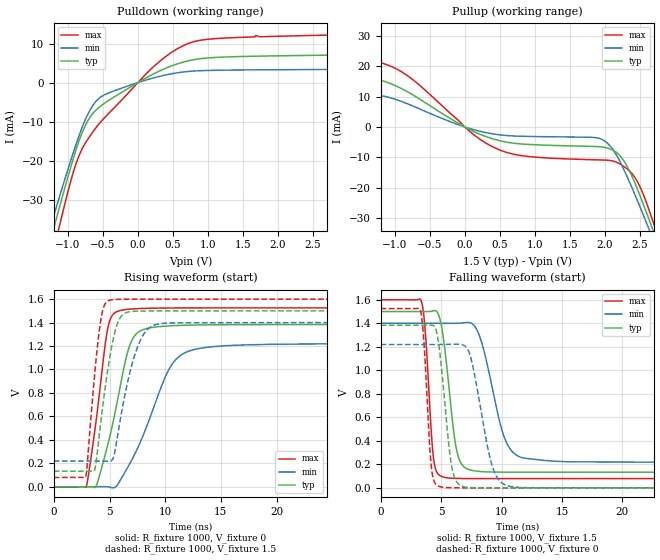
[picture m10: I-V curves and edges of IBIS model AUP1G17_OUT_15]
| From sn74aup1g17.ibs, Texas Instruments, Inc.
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[Model]   AUP1G17_OUT_15
Model_type  Output
Vref =   0
Rref =   1E6
Cref =   30p
Vmeas =   0.75
| variable   typ   min   max
C_comp   2.88pF   2.08pF   4.08pF
| C_pullup   3.12pF   2.08pF   4.08pF
| C_pulldown   2.65pF   2.24pF   3.14pF
[Temperature Range]   40   100   -40
| Ambient temperature   25   85   -40
[Voltage range]   1.5   1.4   1.6
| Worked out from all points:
|   slope of the pulldown table from 0 to 0.225 V, typ, clamps not added: 101 ohm
|   slope of the pullup table from 0 to 0.225 V, typ, clamps not added: 90.4 ohm
|   rising waveform, R_fixture 1000, V_fixture 0: 20-80 % time 1.89ns typ, 3.12ns min, 1.2ns max; typ from 0 V to 1.38 V
|   falling waveform, R_fixture 1000, V_fixture 1.5: 20-80 % time 888ps typ, 1.59ns min, 538ps max; typ from 1.5 V to 0.133 V
|   rising waveform, R_fixture 1000, V_fixture 1.5: 20-80 % time 1.22ns typ, 1.65ns min, 879ps max; typ from 0.133 V to 1.5 V
|   falling waveform, R_fixture 1000, V_fixture 0: 20-80 % time 801ps typ, 1.33ns min, 499ps max; typ from 1.38 V to 0 V
[Pulldown]
| AUP1G17_OUT_15
|   Voltage   I(typ)   I(min)   I(max)
-3.6V     -206.1mA   -188.4mA   -227.8mA
-1.265V   -41.59mA   -37.94mA   -47.65mA
-1.21V    -37.9mA    -34.62mA   -43.48mA
-1.11V    -31.29mA   -28.67mA   -36mA
-945mV    -20.84mA   -19.21mA   -24.37mA
-855mV    -15.7mA    -14.39mA   -19.43mA
-720mV    -9.972mA   -8.297mA   -14.65mA
-570mV    -6.595mA   -4.269mA   -10.91mA
260mV     2.544mA    1.373mA    4.642mA
810mV     5.906mA    2.979mA    10.53mA
1.685V    6.762mA    3.268mA    12.01mA
7.2V      7.827mA    3.609mA    13.77mA
[Pullup]
| AUP1G17_OUT_15
|   Voltage   I(typ)   I(min)   I(max)
-3.6V     29.66mA    17.95mA    40.7mA
-2.925V   22.54mA    13.64mA    31.9mA
-2.13V    15.77mA    9.503mA    23.16mA
-1.025V   13.91mA    9.322mA    19.64mA
130mV     -1.525mA   -910.1uA   -2.565mA
590mV     -4.979mA   -2.819mA   -8.32mA
1.925V    -6.506mA   -3.765mA   -10.85mA
2.175V    -8.513mA   -9.57mA    -11.67mA
2.395V    -16.55mA   -20.31mA   -15.49mA
2.615V    -29.32mA   -32.63mA   -26.15mA
2.72V     -35.89mA   -38.74mA   -33.2mA
7.2V      -352.6mA   -330.3mA   -379.5mA
[Ramp]
| AUP1G17_OUT_15
| variable   typ   min   max
dV/dt_r   0.83/1.91E-09   0.74/3.15E-09   0.92/1.20E-09
dV/dt_f   0.83/8.95E-10   0.71/1.60E-09   0.92/5.43E-10
R_load = 1000
[Rising Waveform]
| AUP1G17_OUT_15
R_fixture =   1000
C_fixture =   0
L_fixture =   0
V_fixture =   0
V_fixture_min = 0
V_fixture_max = 0
|   Time   V(typ)   V(min)   V(max)
0s        16.57nV    92.2nV     986.7pV
2.925ns   299.7uV    -18.59uV   4.96mV
3.795ns   5.632mV    236.3uV    562.4mV
4.78ns    335.2mV    269.9uV    1.318V
5.655ns   706.7mV    9.617mV    1.493V
6.605ns   1.14V      160.7mV    1.513V
7.325ns   1.296V     289.5mV    1.518V
10.25ns   1.371V     984mV      1.524V
11.9ns    1.378V     1.148V     1.525V
34.99ns   1.383V     1.22V      1.525V
[Falling Waveform]
| AUP1G17_OUT_15
R_fixture =   1000
C_fixture =   0
L_fixture =   0
V_fixture =   1.5
V_fixture_min = 1.4
V_fixture_max = 1.6
|   Time   V(typ)   V(min)   V(max)
0s        1.5V       1.4V       1.6V
3.365ns   1.5V       1.4V       1.588V
3.69ns    1.499V     1.4V       1.327V
4.355ns   1.506V     1.4V       268.4mV
5.025ns   1.379V     1.4V       97.91mV
6.225ns   353.7mV    1.399V     80.35mV
7.21ns    159.4mV    1.408V     79.29mV
10.26ns   133.6mV    422.5mV    79.08mV
11.49ns   133.3mV    264.4mV    79.08mV
34.99ns   133.1mV    219.3mV    79.08mV
[Rising Waveform]
| AUP1G17_OUT_15
R_fixture =   1000
C_fixture =   0
L_fixture =   0
V_fixture =   1.5
V_fixture_min = 1.4
V_fixture_max = 1.6
|   Time   V(typ)   V(min)   V(max)
0s        133.1mV    219.3mV    79.08mV
2.855ns   133.3mV    219.4mV    81.83mV
3.655ns   141.8mV    219.5mV    944.3mV
4.09ns    446.9mV    219.4mV    1.335V
4.92ns    1.044V     217.5mV    1.588V
5.39ns    1.282V     261.6mV    1.596V
6.075ns   1.456V     629.7mV    1.599V
7.455ns   1.497V     1.175V     1.6V
8.935ns   1.499V     1.376V     1.6V
34.99ns   1.5V       1.4V       1.6V
[Falling Waveform]
| AUP1G17_OUT_15
R_fixture =   1000
C_fixture =   0
L_fixture =   0
V_fixture =   0
V_fixture_min = 0
V_fixture_max = 0
|   Time   V(typ)   V(min)   V(max)
0s        1.383V     1.22V      1.525V
3.28ns    1.383V     1.22V      1.511V
4.18ns    1.385V     1.22V      191.1mV
4.78ns    1.237V     1.22V      14.86mV
5.83ns    212.8mV    1.221V     826.9uV
6.7ns     15.21mV    1.219V     87.08uV
7.515ns   2.208mV    1.083V     13.95uV
9.225ns   100.5uV    187.3mV    1.044uV
10.34ns   23.19uV    23.19mV    304.8nV
34.99ns   -57.37nV   16.27nV    -77.7nV
